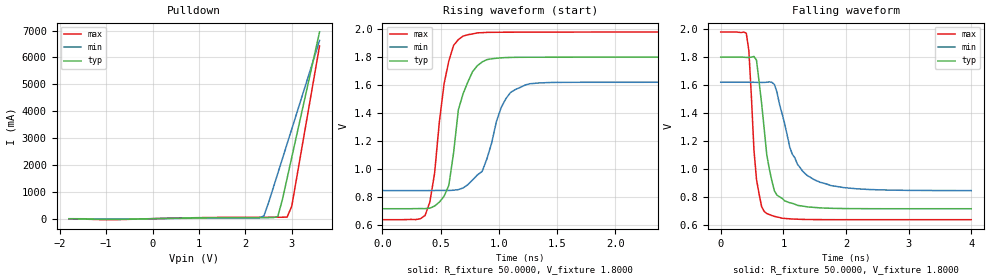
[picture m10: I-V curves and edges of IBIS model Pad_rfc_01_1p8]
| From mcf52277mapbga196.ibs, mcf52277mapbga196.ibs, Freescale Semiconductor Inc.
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|   Model Pad_rfc_01_1p8
[Model]   Pad_rfc_01_1p8
Model_type   Open_drain
Polarity   Non-Inverting
Enable   Active-High
Vmeas =   0.9000V
C_comp   1.7450pF   1.6200pF   1.8900pF
[Temperature Range]   25.0000   0.1500k   -40.0000
[Voltage Range]   1.8000V   1.6200V   1.9800V
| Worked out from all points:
|   slope of the pulldown table from 0 to 0.27 V, typ, clamps not added: 28.5 ohm
|   rising waveform, R_fixture 50.0000, V_fixture 1.8000: 20-80 % time 136ps typ, 172ps min, 120ps max; typ from 0.714 V to 1.8 V
|   falling waveform, R_fixture 50.0000, V_fixture 1.8000: 20-80 % time 185ps typ, 345ps min, 113ps max; typ from 1.8 V to 0.714 V
[Pulldown]
| voltage   I(typ)   I(min)   I(max)
-1.8V     -2.83mA    -1.394mA   -5.24mA
-900mV    -27.33mA   -13.6mA    -36.25mA
900mV     25.68mA    16.19mA    35.07mA
2.3V      37.56mA    28.04mA    53.29mA
2.4V      37.73mA    104mA      53.51mA
2.5V      37.9mA     590mA      53.71mA
2.6V      38.94mA    1.139A     53.89mA
2.7V      83.53mA    1.687A     54.06mA
2.8V      719.2mA    2.236A     54.24mA
2.9V      1.498A     2.784A     58.2mA
3V        2.276A     3.333A     458.6mA
3.6V      6.949A     6.633A     6.432A
[Ramp]
| variable   typ   min   max
dV/dt_r   0.6515/0.1383n   0.4655/0.1931n   0.8066/0.1109n
dV/dt_f   0.6516/0.1706n   0.4655/0.3220n   0.8066/0.1060n
R_load = 50.0000
[Rising Waveform]
R_fixture = 50.0000
V_fixture = 1.8000
V_fixture_min = 1.6200
V_fixture_max = 1.9800
| time   V(typ)   V(min)   V(max)
0s        714.1mV    844.1mV    635.7mV
367.3ps   714.9mV    844mV      665.8mV
449ps     733.5mV    844.6mV    969.8mV
530.6ps   804mV      844.7mV    1.611V
571.4ps   882.8mV    844.7mV    1.773V
693.9ps   1.538V     862.8mV    1.95V
857.1ps   1.765V     981mV      1.975V
1.061ns   1.797V     1.503V     1.978V
1.265ns   1.799V     1.609V     1.979V
4ns       1.8V       1.62V      1.98V
[Falling Waveform]
R_fixture = 50.0000
V_fixture = 1.8000
V_fixture_min = 1.6200
V_fixture_max = 1.9800
| time   V(typ)   V(min)   V(max)
0s        1.8V       1.62V      1.98V
408.2ps   1.798V     1.62V      1.972V
449ps     1.797V     1.62V      1.847V
530.6ps   1.805V     1.62V      1.135V
571.4ps   1.778V     1.619V     923.4mV
734.7ps   1.102V     1.62V      679.9mV
898ps     811.7mV    1.549V     654.7mV
1.143ns   752.9mV    1.105V     640.5mV
1.469ns   724.4mV    928.1mV    636.6mV
4ns       714.1mV    844.2mV    635.7mV
